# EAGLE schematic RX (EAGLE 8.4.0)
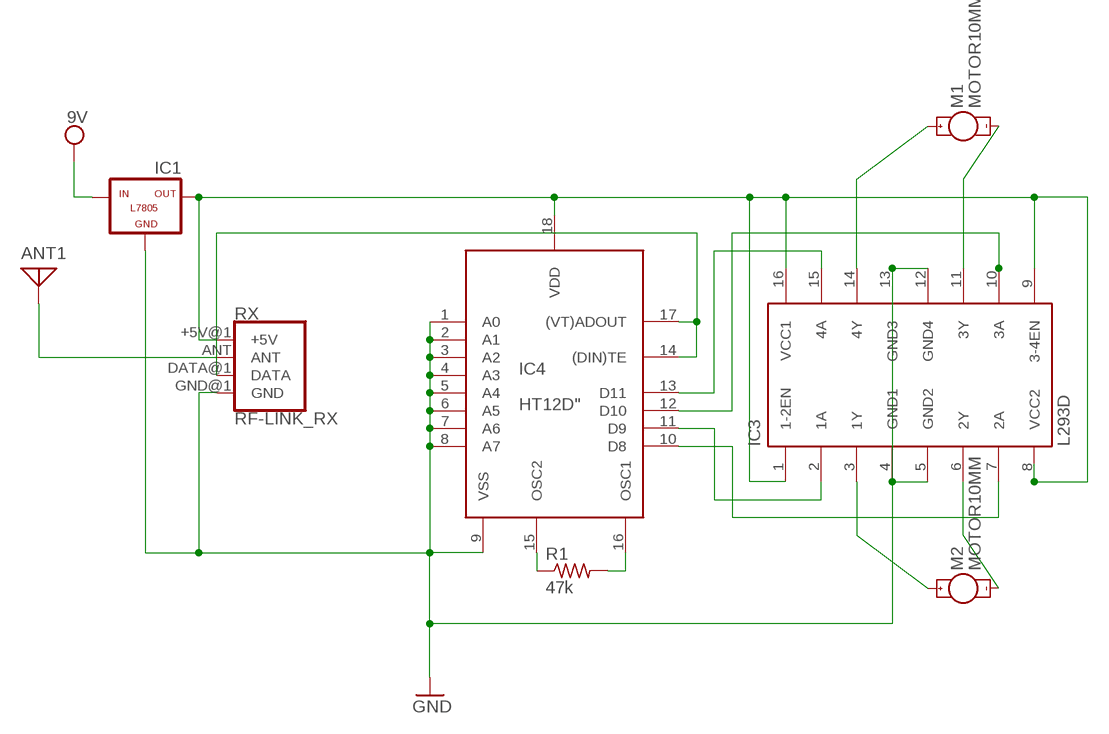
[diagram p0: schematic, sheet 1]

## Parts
ANT1  ANTENNA  [PAD-01]
IC1  5V  L7805  [78XXL]
IC3  L293D  [DIL16]
IC4  HT12D"  [18-DIP-A]
M1  MOTOR10MM  [VIBE-MOTOR-10MM]
M2  MOTOR10MM  [VIBE-MOTOR-10MM]
R1  47k  R-US_R0201  [R0201]
RX  RF-LINK_RX  [RF-LINK_RX]

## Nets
N$1: IC3.6(2Y) M2.-
N$2: ANT1.1 RX.ANT
N$3: IC3.10(3A) IC4.12(D10)
N$4: IC3.11(3Y) M1.-
N$5: IC4.15(OSC2) R1.1
N$6: IC4.16(OSC1) R1.2
N$8: IC4.14((DIN)TE) IC4.17((VT)ADOUT) RX.DATA@1(DATA)
N$9: IC1.OUT IC3.1(1-2EN) IC3.8(VCC2) IC3.9(3-4EN) IC3.16(VCC1) IC4.18(VDD) RX.+5V@1(+5V)
N$11: IC3.7(2A) IC4.10(D8)
N$12: IC3.2(1A) IC4.11(D9)
N$13: IC3.14(4Y) M1.+
N$14: IC3.15(4A) IC4.13(D11)
N$15: IC3.3(1Y) M2.+
VSS: IC1.GND IC1.IN IC3.4(GND1) IC3.5(GND2) IC3.12(GND4) IC3.13(GND3) IC4.1(A0) IC4.2(A1) IC4.3(A2) IC4.4(A3) IC4.5(A4) IC4.6(A5) IC4.7(A6) IC4.8(A7) IC4.9(VSS) RX.GND@1(GND) ; supply symbol labelled 9V, GND

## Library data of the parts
ANT1 = discrete:ANTENNA: Antenna
IC1 = l7805:L7805: VOLTAGE REGULATOR
IC3 = st-microelectronics:L293D: PUSH-PULL 4 CHANNEL DRIVER; MPN: L293D; OC_FARNELL: 9589619; OC_NEWARK: 56P8249
IC4 = holtek:HT12D: decoder = receiver ic
M1 M2 = SparkFun-Electromechanical:MOTOR: Motor (Single-Phase); PROD_ID: COMP-08572; SF_SKU: ROB-08449
R1 = rcl:R-US_: RESISTOR, American symbol
RX = SparkFun-RF:RF-LINK_RX: RF Link Receiver (434 MHz, 315 MHz) These wireless receivers work with equivalent transmitters. They can easily fit into a breadboard and work well with microcontrollers to create a very simple wireless data link. Since these are only receivers, they will only work communicating data one-way, you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; SF_ID: WRL-10533

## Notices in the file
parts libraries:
SparkFun-RF: Licensing: Creative Commons ShareAlike 4.0 International - https://creativecommons.org/licenses/by-sa/4.0
